|Texas Instruments Incorporated
| Quad 14-Bit High Accuracy +/-15 V Output Serial Input Digital-To-Analog
| Converter
| Marketing part#   Digital Voltage Range   Package-type   #pins
|  DAC8234SPFB   1.7V to 5.5V   TQFP   48
|  DAC8234SPFBR   1.7V to 5.5V   TQFP   48
|  DAC8234SRHAR   1.7V to 5.5V   VQFN   40
|  DAC8234SRHAT   1.7V to 5.5V   VQFN   40
[IBIS Ver]   3.2
[File name]   dac8234.ibs
|SIMDE Ver   V2.0 - 201002 - RHL4 - Build 372
[File Rev]   1.0
[Date]   12/02/2010
[Source]
| Texas Instruments Incorporated.
| Analog-eLab Design Center, HPA
| 12500 TI Blvd
| Dallas, TX -75243
| e-mail: elab_ibis@list.ti.com
| -Model generated from simulations in TISPICE
[Notes]   Revision History:
|   DAC8234 is a relative part of DAC7716.
|   Rev 1.0: 12/02/2010
|   - Initial version of the model
|   - Model generated from simulations in TISPICE
|   - Model matched to SPICE simulation
|   - C_comp although listed in numerical order of value are
|   obtained from varying PVT conditions. For PVT conditions for
|   each specific value refer the buffer description under
|   respective [Model]. IBIS model user is responsible for using
|   appropriate C_comp to simulate for Signal Integrity.
[Disclaimer]
| This model is designed as an aid for customers of Texas Instruments.
| TI and its licensors and suppliers make no warranties, either expressed
| or implied, with respect to this  model, including the warranties of
| merchantability or fitness for a particular purpose. The model is
| provided solely on an "as is" basis. The entire risk as to its quality
| and performance is with the customer.
[Copyright]
 (C) Copyright 2010 Texas Instruments Incorporated.All rights reserved.
|   DAC8234SPFB
[Component]   DAC8234SPFB
[Manufacturer]   TI
[Package]   |48 TQFP - PFB package
|   typ   min   max
R_pkg   0.05575   0.05233   0.06123
L_pkg   2.3935nH   2.19243nH   3.0931nH
C_pkg   0.46377pF   0.39575pF   0.56778pF
[Pin]  signal_name   model_name   R_pin   L_pin   C_pin
1   NC   NC   0.00846   1.89714nH  0.46999pF
2   CS   INPUT   0.05268   2.38048nH  0.48539pF
3   SCLK   INPUT   0.05233   2.33241nH  0.47156pF
4   SDI   INPUT   0.05299   2.35660nH  0.46932pF
5   SDO   TRI-STATE   0.05296   2.19873nH  0.42669pF
6   LDAC   INPUT   0.05362   2.19243nH  0.39575pF
7   RST   INPUT   0.05384   2.19750nH  0.39705pF
8   GPIO-0   IO   0.05379   2.22104nH  0.42959pF
9   GPIO-1   IO   0.05462   2.40269nH  0.47222pF
10   UNI/BIP-A   INPUT_MODE   0.05422   2.38457nH  0.47518pF
11   DGND   GND   0.05535   2.45357nH  0.49328pF
12   NC   NC   0.00839   1.88607nH  0.47744pF
13   IOVDD   POWER   0.06115   3.11193nH  0.55903pF
14   DVDD   POWER   0.05704   2.50809nH  0.49525pF
15   VOUT-0   TERM   0.05517   2.41766nH  0.47916pF
16   RFB2-0   TERM   0.05504   2.41774nH  0.48100pF
17   RFB1-0   TERM   0.05575   2.28063nH  0.44102pF
18   SGND-0   GND   0.03272   2.06959nH  0.44901pF
19   NC   NC   0.00547   1.10876nH  0.30844pF
20   SGND-1   GND   0.03030   1.96012nH  0.46897pF
21   RFB1-1   TERM   0.05572   2.43629nH  0.48299pF
22   RFB2-1   TERM   0.05722   2.47251nH  0.48113pF
23   VOUT-1   TERM   0.05693   2.50187nH  0.49207pF
24   NC   NC   0.00841   1.89099nH  0.47397pF
25   NC   NC   0.00846   1.89714nH  0.46999pF
26   AVDD   POWER   0.03198   2.15470nH  0.53414pF
27   AGND   GND   0.05949   2.53061nH  0.48305pF
28   AVSS   GND   0.06076   2.57180nH  0.48545pF
29   REFGND-A   TERM   0.05860   2.35433nH  0.44001pF
30   REF-A   TERM   0.05846   2.32563nH  0.40835pF
31   REF-B   TERM   0.05721   2.28920nH  0.40637pF
32   REFGND-B   TERM   0.05639   2.29064nH  0.43703pF
33   AVSS   GND   0.05681   2.45949nH  0.48203pF
34   VMON   TERM   0.05831   2.49187nH  0.49022pF
35   AVDD   POWER   0.03251   2.13344nH  0.55407pF
36   NC   NC   0.00839   1.88607nH  0.47744pF
37   NC   NC   0.00847   1.89920nH  0.46872pF
38   VOUT-3   TERM   0.05711   2.49794nH  0.48973pF
39   RFB2-3   TERM   0.05739   2.46568nH  0.48183pF
40   RFB1-3   TERM   0.05588   2.42915nH  0.48253pF
41   SGND-3   GND   0.03039   1.95775nH  0.46837pF
42   NC   NC   0.00549   1.11031nH  0.30811pF
43   SGND-2   GND   0.03279   2.03644nH  0.44937pF
44   RFB1-2   TERM   0.05590   2.27123nH  0.44105pF
45   RFB2-2   TERM   0.05521   2.41018nH  0.47957pF
46   VOUT-2   TERM   0.05532   2.40768nH  0.48060pF
47   AIN   TERM   0.05723   2.49745nH  0.50032pF
48   UNI/BIP-B   INPUT_MODE   0.06123   3.09310nH  0.56778pF
|   DAC8234SRHA
[Component]   DAC8234SRHA
[Manufacturer]   TI
[Package]   |40 VQFN - RHA package
|   typ   min   max
R_pkg   0.04602   0.04063   0.05300
L_pkg   1.06961nH   0.93212nH   1.25554nH
C_pkg   0.13028pF   0.11935pF   0.14555pF
[Pin]  signal_name   model_name   R_pin   L_pin   C_pin
1   CS   INPUT   0.04680   1.09784nH  0.12009pF
2   SCLK   INPUT   0.04338   1.00441nH  0.12564pF
3   SDI   INPUT   0.04205   0.96892nH  0.12192pF
4   SDO   TRI-STATE   0.04087   0.93842nH  0.11975pF
5   LDAC   INPUT   0.04063   0.93212nH  0.11935pF
6   RST   INPUT   0.04144   0.95288nH  0.12136pF
7   GPIO-0   IO   0.04349   1.00635nH  0.12578pF
8   GPIO-1   IO   0.04636   1.08227nH  0.13102pF
9   UNI/BIP-A   INPUT_MODE   0.04835   1.13584nH  0.13570pF
10   DGND   GND   0.05219   1.24193nH  0.12957pF
11   IOVDD   POWER   0.04702   1.10244nH  0.11936pF
12   DVDD   POWER   0.04466   1.03549nH  0.12871pF
13   VOUT-0   TERM   0.04249   0.97587nH  0.12568pF
14   RFB2-0   TERM   0.04347   0.99937nH  0.12872pF
15   RFB1-0   TERM   0.04755   1.10606nH  0.13984pF
16   SGND-0   GND   0.02630   0.92116nH  0.18075pF
17   SGND-1   GND   0.02173   0.69725nH  0.16050pF
18   RFB1-1   TERM   0.04594   1.06367nH  0.13573pF
19   RFB2-1   TERM   0.05163   1.21544nH  0.14351pF
20   VOUT-1   TERM   0.05290   1.25273nH  0.13013pF
21   AVDD   POWER   0.02529   0.77493nH  0.17375pF
22   AGND   GND   0.05413   1.28284nH  0.14465pF
23   AVSS   GND   0.05366   1.26967nH  0.14583pF
24   REFGND-A   TERM   0.04858   1.13191nH  0.13706pF
25   REF-A   TERM   0.04606   1.06406nH  0.13183pF
26   REF-B   TERM   0.04377   1.00296nH  0.12714pF
27   REFGND-B   TERM   0.04390   1.00672nH  0.12759pF
28   AVSS   GND   0.04663   1.07967nH  0.13522pF
29   VMON   TERM   0.05220   1.23054nH  0.14555pF
30   AVDD   POWER   0.02609   0.86788nH  0.17062pF
31   VOUT-3   TERM   0.05300   1.25554nH  0.12972pF
32   RFB2-3   TERM   0.05174   1.21844nH  0.14368pF
33   RFB1-3   TERM   0.04606   1.06707nH  0.13598pF
34   SGND-3   GND   0.02180   0.70038nH  0.16086pF
35   SGND-2   GND   0.02635   0.92416nH  0.18103pF
36   RFB1-2   TERM   0.04767   1.10926nH  0.14007pF
37   RFB2-2   TERM   0.04360   1.00298nH  0.12901pF
38   VOUT-2   TERM   0.04263   0.97956nH  0.12622pF
39   AIN   TERM   0.04486   1.04084nH  0.12947pF
40   UNI/BIP-B   INPUT_MODE   0.04719   1.10713nH  0.12029pF
41   ThermalPAD   GND   0.00002   0.01121nH  0.15552pF
|   Model Selectors
[Model Selector]  INPUT
INPUT_1p8   1.8V digital input
INPUT_3p3   3.3V digital input
INPUT_5   5.0V digital input
|NOTES   Model INPUT_EN split into three Models INPUT_1p8 INPUT_3p3
|   and INPUT_5 to accomodate voltage range of 1.7V - 5.5V
|   INPUT_1p8 operates in voltage range of 1.7 - 1.8 - 1.9
|   INPUT_3p3 operates in voltage range of 3.0 - 3.3 - 3.6
|   INPUT_5 operates in voltage range of 4.5 - 5.0 - 5.5
|   The min pin frequency for Model INPUT is 50MHz
|   This is referenced with datasheet
[Model Selector]  INPUT_MODE
INPUT_AIN_1p8_MODE0  1.8V digital input
INPUT_AIN_3p3_MODE0  3.3V digital input
INPUT_AIN_5_MODE0   5.0V digital input
|NOTES   Model INPUT_MODE split into three Models INPUT_1p8_MODE0,
|   INPUT_3p3_MODE0,INPUT_5_MODE0 to accomodate voltage range
|   of 1.7V - 5.5V. INPUT_1p8_MODE0 operates in voltage range of
|   1.7-1.8-1.9. INPUT_3p3_MODE0 operates in voltage range of
|   3 - 3.3 - 3.6. INPUT_5_MODE0 operates in voltage range of
|   4.5 - 5 - 5.5. The max pin frequency for Model INPUT_MODE
|   is 50MHz.
[Model Selector]  TRI-STATE
TRI_1p8   1.8V digital tri-state output
TRI_3p3   3.3V digital tri-state output
TRI_5   5.0V digital tri-state output
|NOTES   Model TRI-STATE split into three Models TRI_1p8, TRI_3p3
|   and TRI_5 to accomodate voltage range of 1.7V - 5.5V
|   TRI_1p8 operates in voltage range of 1.7 - 1.8 - 1.9
|   TRI_3p3 operates in voltage range of 3.0 - 3.3 - 3.6
|   TRI_5 operates in voltage range of 4.5 - 5.0 - 5.5
|   The max pin frequency for Model TRI-STATE is 12.5MHz
|   This is referenced with datasheet
[Model Selector]  IO
IO_1p8   1.8V digital io
IO_3p3   3.3V digital io
IO_5   5.0V digital io
|NOTES   Model IO split into three Models IO_1p8, IO_3p3
|   and IO_5 to accomodate voltage range of 1.7V - 5.5V
|   IO_1p8 operates in voltage range of 1.7 - 1.8 - 1.9
|   IO_3p3 operates in voltage range of 3.0 - 3.3 - 3.6
|   IO_5 operates in voltage range of 4.5 - 5.0 - 5.5
|   The min pin frequency for Model IO is 0.5MHz
[Model selector] TERM
 TERM_1p8  1.8V nominal termination
 TERM_3p3  3.3V nominal termination
 TERM_5   5.0V nominal termination
|   Termination - TERM_3p3
[Model] TERM_3p3
Model_type Terminator
C_comp   1.0e-20F  1.0e-20F  1.0e-20F
| variable   typ   min   max
[Voltage Range]   3.30000v  3.00000V  3.60000V
[POWER Clamp Reference]  3.30000v  3.00000V  3.60000V
[GND Clamp Reference]   0.00000V  0.00000V  0.00000V
|Ambient Temperature   25   105   -40
|Junction Temperature
[Temperature Range]   42   122   -40
|   Termination - TERM_5
[Model] TERM_5
Model_type Terminator
C_comp   1.0e-20F  1.0e-20F  1.0e-20F
| variable   typ   min   max
[Voltage Range]   5.00000V  4.50000V  5.50000V
[POWER Clamp Reference]  5.00000V  4.50000V  5.50000V
[GND Clamp Reference]   0.00000V  0.00000V  0.00000V
|Ambient Temperature   25   105   -40
|Junction Temperature
[Temperature Range]   42   122   -40
|   Termination - TERM_1p8
[Model] TERM_1p8
Model_type Terminator
C_comp   1.0e-20F  1.0e-20F  1.0e-20F
| variable   typ   min   max
[Voltage Range]   1.80000v  1.70000V  1.90000V
[POWER Clamp Reference]  1.80000v  1.70000V  1.90000V
[GND Clamp Reference]   0.00000V  0.00000V  0.00000V
|Ambient Temperature   25   105   -40
|Junction Temperature
[Temperature Range]   42   122   -40
| Models and submodels in the file (15): INPUT_1p8 (Input), INPUT_3p3 (Input), INPUT_5 (Input), INPUT_AIN_1p8_MODE0 (Input), INPUT_AIN_3p3_MODE0 (Input), INPUT_AIN_5_MODE0 (Input), TRI_1p8 (3-state), TRI_3p3 (3-state), TRI_5 (3-state), IO_1p8 (I/O_open_drain), IO_3p3 (I/O_open_drain), IO_5 (I/O_open_drain), TERM_3p3 (Terminator), TERM_5 (Terminator), TERM_1p8 (Terminator)
